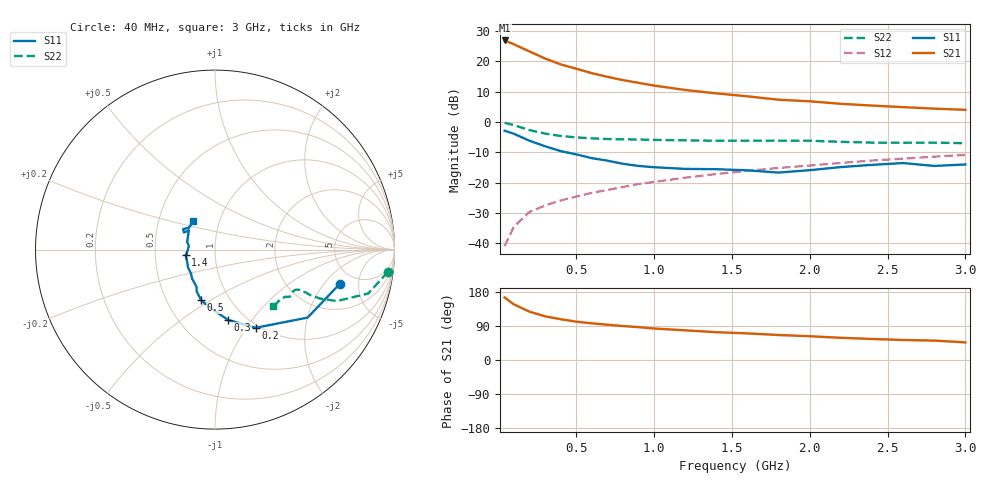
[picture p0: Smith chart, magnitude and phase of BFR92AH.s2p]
! Filename:  BFR92AH.S2P  Version:  2.0
! Philips part #: BFR92A  Date: May 1990
! Bias condition: Vce=10V, Ic=10mA
#  MHz  S  MA  R  50
! Freq  S11  S21  S12  S22  !GUM [dB]
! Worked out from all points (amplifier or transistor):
!   21 points, 40 MHz to 3 GHz, reference 50 ohm
!   highest |S21| = 26.9 dB at 40 MHz (marker M1)
!   |S21| within 3 dB of that: start of sweep to 173.5 MHz
!   unconditionally stable (mu >= 1): 995.6 MHz to 2.477 GHz
!   at 300 MHz: K = 0.69, MSG = 24.2 dB, |S12| = -27.5 dB
!   at 1 GHz: K = 1.00, MAG = 15.7 dB, |S12| = -19.7 dB
!   at 3 GHz: K = 0.99, MSG = 7.4 dB, |S12| = -10.8 dB
!   S11 on the Smith chart (normalised r, x): 40 MHz: 3.68, -2.94; 200 MHz: 0.96, -1.11; 300 MHz: 0.83, -0.78; 500 MHz: 0.74, -0.46; 1.4 GHz: 0.72, -0.04; 3 GHz: 0.75, +0.25
40  0.72 -15.5  22.11 164.9  0.009 84.4  0.971 -7.4
100  0.64 -36.3  19.09 146.7  0.019 71.8  0.888 -16.0
200  0.491 -62.5  14.57 127.5  0.033 66.9  0.737 -22.9
300  0.399 -79.3  11.15 115.3  0.042 66.2  0.645 -25.0
400  0.332 -93.0  8.913 107.6  0.051 66.1  0.59 -25.5
500  0.293 -105.2  7.577 101.1  0.059 67.9  0.558 -25.3
600  0.254 -113.7  6.396 96.8  0.068 69.1  0.539 -25.5
700  0.231 -116.5  5.558 93.2  0.076 70.7  0.525 -25.5
800  0.205 -128.9  4.91 89.6  0.085 71.8  0.519 -25.5
900  0.189 -134.8  4.431 86.7  0.095 72.5  0.516 -25.8
1000  0.18 -146.7  3.989 83.1  0.103 72.7  0.508 -26.0
1200  0.169 -156.5  3.375 78.3  0.121 73.5  0.499 -26.8
1400  0.167 -169.7  2.967 73.4  0.139 73.3  0.492 -28.7
1600  0.16 -171.2  2.653 70.2  0.157 73.9  0.493 -29.7
1800  0.147 172.2  2.333 65.9  0.175 73.2  0.493 -31.2
2000  0.161 164.3  2.197 62.7  0.192 73.1  0.492 -32.4
2200  0.181 143.5  1.998 58.6  0.212 73.0  0.472 -33.8
2400  0.197 151.3  1.868 55.5  0.232 71.9  0.458 -37.1
2600  0.211 147.3  1.76 52.8  0.249 71.1  0.455 -40.6
2800  0.189 139.6  1.663 51.2  0.269 71.0  0.458 -42.8
3000  0.2 128.0  1.591 46.5  0.287 69.7  0.448 -44.1
